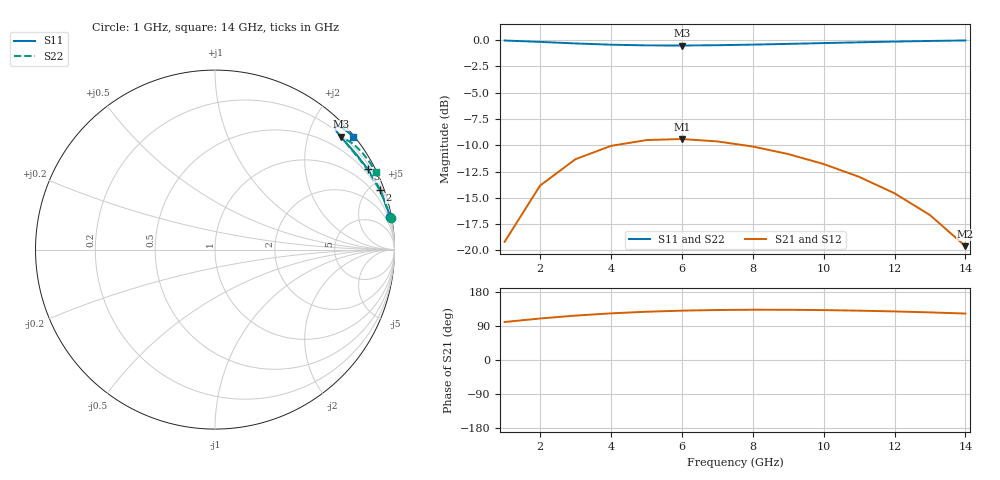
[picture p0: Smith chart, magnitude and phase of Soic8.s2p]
# GHZ S RI R 50
!Output file by EM3DS_5.0
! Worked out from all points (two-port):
!   14 points, 1 GHz to 14 GHz, reference 50 ohm
!   highest |S21| = -9.41 dB at 6 GHz (marker M1); lowest = -19.6 dB at 14 GHz (marker M2)
!   |S21| within 3 dB of the highest: 2.567 GHz to 10.51 GHz (7.946 GHz wide, 121 % of centre)
!   lowest |S11| = -0.5 dB at 6 GHz (marker M3), VSWR 32.91, Z = 11.8 + j130 ohm
!   |S11| at or under -10 dB: nowhere
!   |S22| runs from -0.5 to 0.0 dB; largest |S21 - S12| = 3.7e-15
!   S11 on the Smith chart (normalised r, x): 1 GHz: 0, +11; 2 GHz: 0.35, +5.68; 3 GHz: 0.33, +4.01; 14 GHz: 0.02, +2.80
1  0.9775 0.1801  -0.0196 0.1082  -0.0196 0.1082  0.9787 0.1736
2  0.9206 0.3333  -0.0679 0.1916  -0.0679 0.1916  0.9252 0.3206
3  0.8512 0.4491  -0.124 0.2415  -0.124 0.2415  0.8611 0.4299
4  0.787 0.5312  -0.1713 0.263  -0.1713 0.263  0.8039 0.5052
5  0.7361 0.5884  -0.203 0.2659  -0.203 0.2659  0.7616 0.5551
6  0.7004 0.6285  -0.2186 0.2583  -0.2186 0.2583  0.7357 0.5867
7  0.6788 0.6562  -0.2203 0.2452  -0.2203 0.2452  0.725 0.6048
8  0.6693 0.6744  -0.2112 0.2293  -0.2112 0.2293  0.7271 0.6116
9  0.67 0.6846  -0.194 0.2116  -0.194 0.2116  0.74 0.6083
10  0.6789 0.6876  -0.1712 0.1922  -0.1712 0.1922  0.7614 0.595
11  0.6947 0.6836  -0.1445 0.1709  -0.1445 0.1709  0.7894 0.5716
12  0.7159 0.6727  -0.1156 0.1469  -0.1156 0.1469  0.8223 0.5375
13  0.7412 0.6549  -0.0858 0.1197  -0.0858 0.1197  0.8581 0.4919
14  0.7696 0.6299  -0.0564 0.0883  -0.0564 0.0883  0.8949 0.4338
